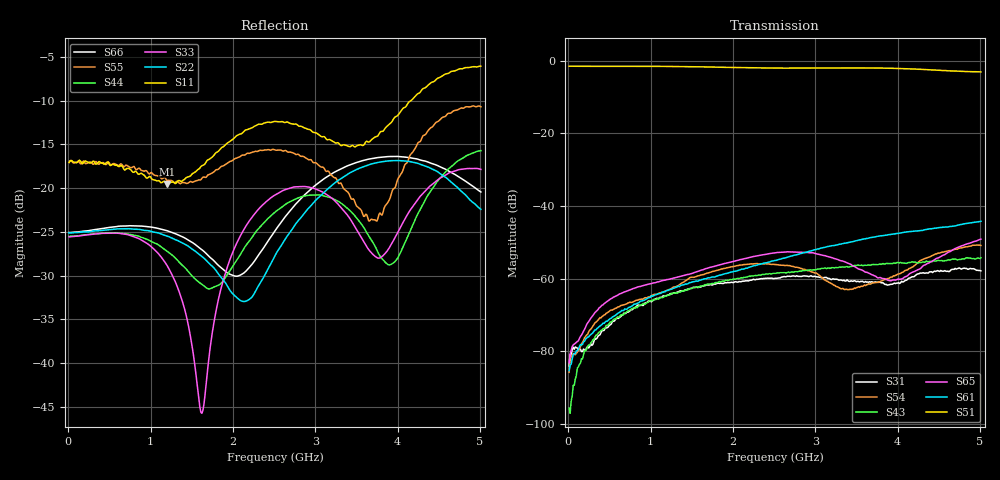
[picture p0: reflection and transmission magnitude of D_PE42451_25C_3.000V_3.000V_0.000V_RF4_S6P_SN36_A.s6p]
! Device ID: PE42451
! Serial: 36
! Insertion: A
! Temp: 25C
! VDD: 3.000
! Control_Hi: 100.000
! Control_Lo: 0.000
! Logic State: RF4
! Port 1: RFC
! Port 2: RF1
! Port 3: RF2
! Port 4: RF3
! Port 5: RF4
! Port 6: RF5
! V1 = 0.00
! V2 = 0.00
! V3 = 3.00
! V4 = 0.00
! IDD: 1.320850e-05
#  Hz  S  RI  R  50
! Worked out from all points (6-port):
!   401 points, 10 MHz to 5.01 GHz, reference 50 ohm
!   strongest paths, dB at 10 MHz, 1.26 GHz, 2.51 GHz, 3.76 GHz, 5.01 GHz:
!     S51: -1.5, -1.5, -2.0, -2.0, -3.0
!     S61: -85.3, -62.9, -55.0, -48.3, -44.2
!     S65: -83.2, -60.0, -52.9, -59.8, -49.1
!     S43: -95.7, -64.0, -58.6, -56.1, -54.3
!     S54: -85.8, -62.6, -56.1, -61.0, -50.8
!     S31: -84.0, -64.2, -59.9, -61.0, -57.8
!   lowest |S11| = -19.5 dB at 1.198 GHz (marker M1), VSWR 1.24, Z = 55.7 - j9.66 ohm
!   |S11| at or under -10 dB: start of sweep to 4.162 GHz
